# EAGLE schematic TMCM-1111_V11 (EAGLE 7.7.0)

## Sheet 1 of 5: CPU
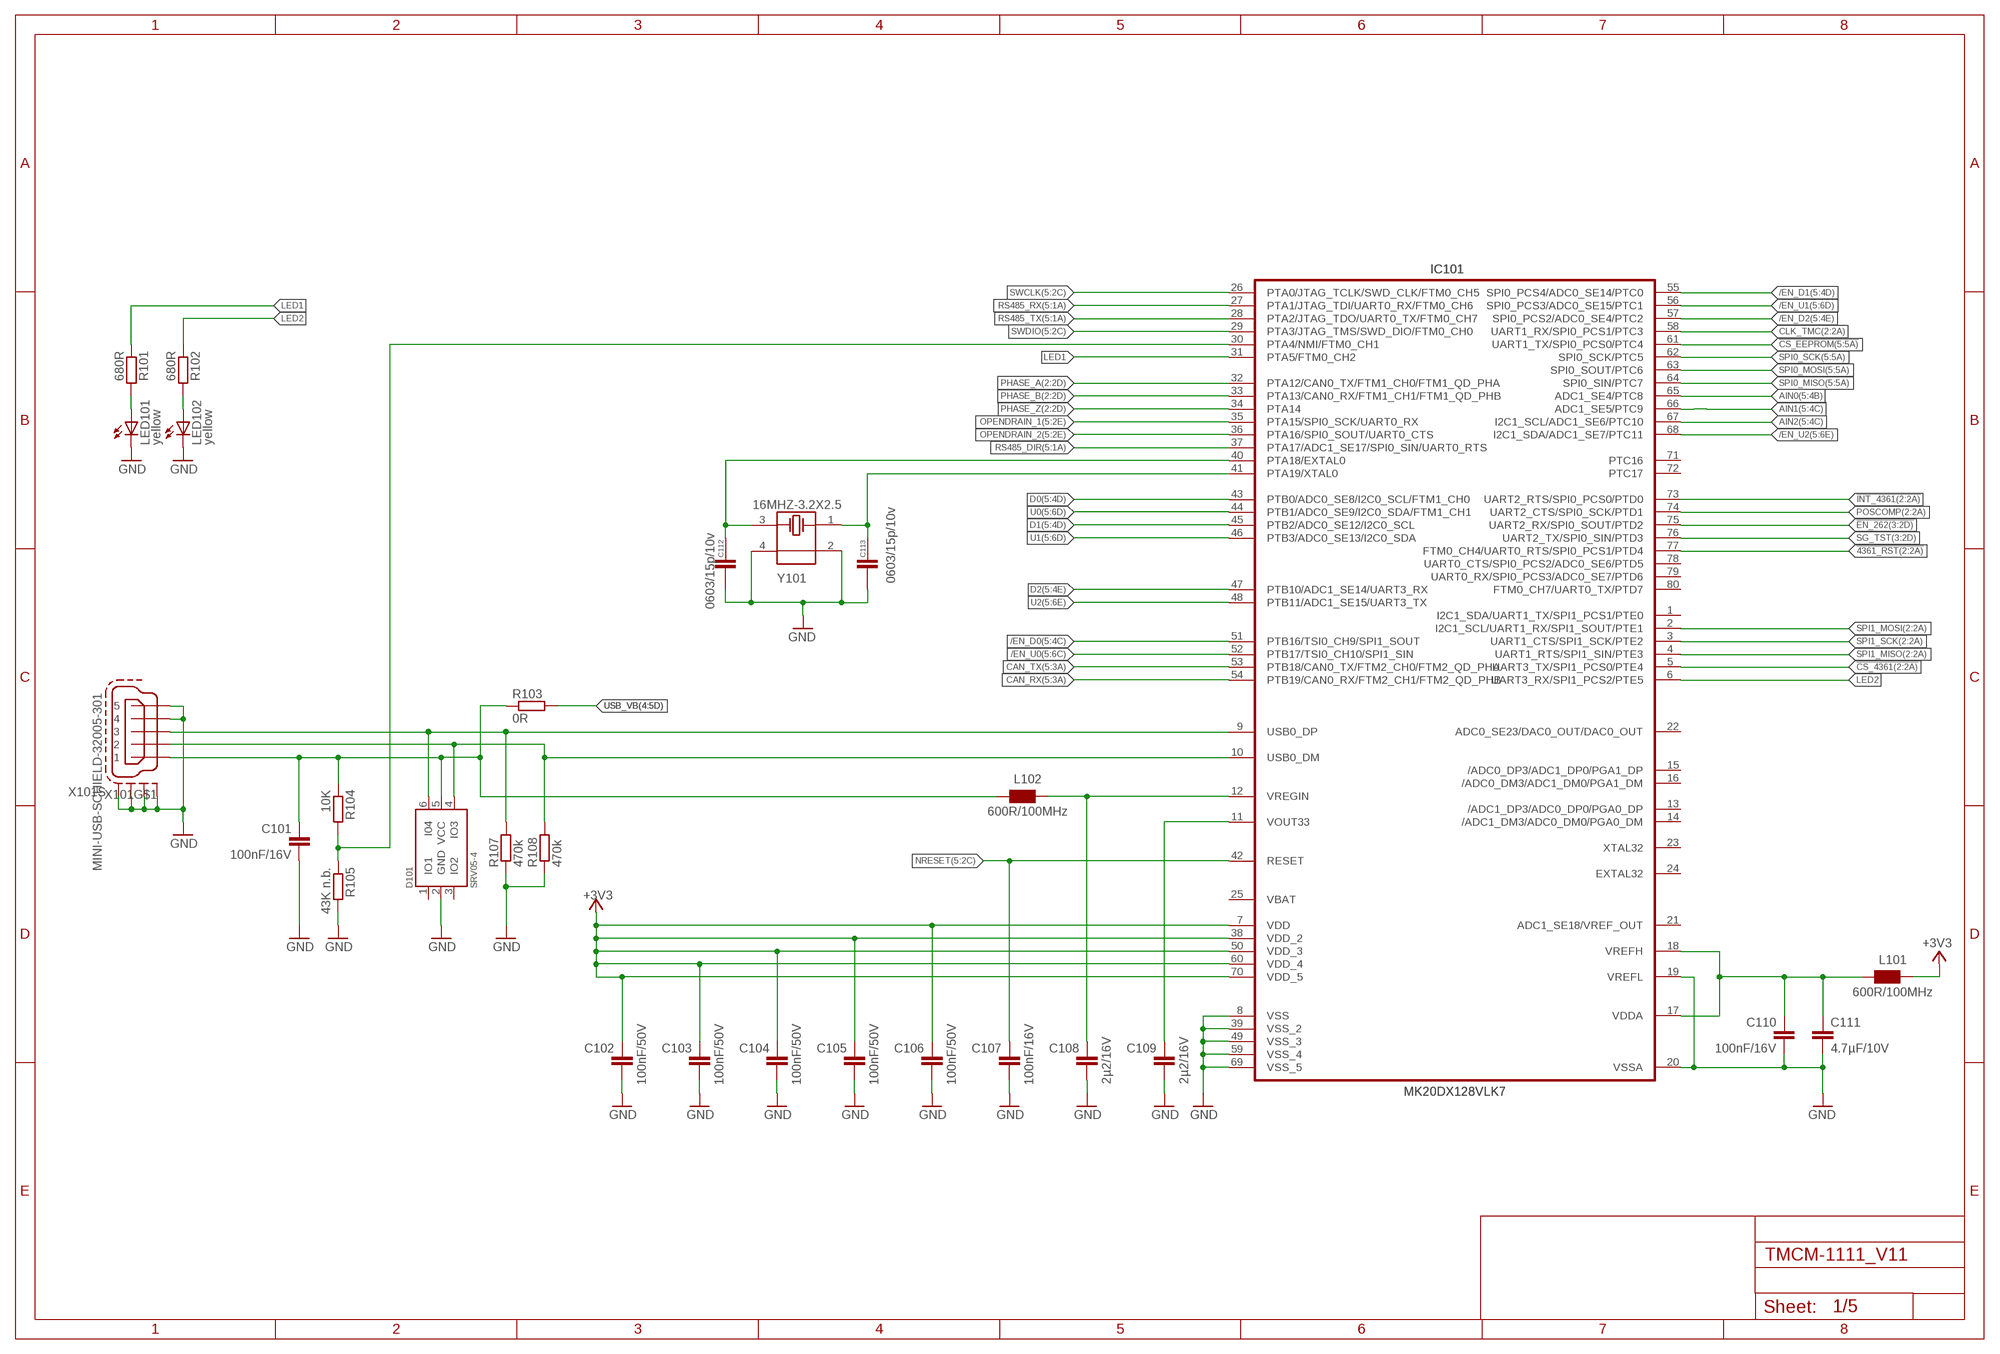
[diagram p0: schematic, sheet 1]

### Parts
C101  100nF/16V  C-EUC0603  [C0603]
C102  100nF/50V  C-EUC0603  [C0603]
C103  100nF/50V  C-EUC0603  [C0603]
C104  100nF/50V  C-EUC0603  [C0603]
C105  100nF/50V  C-EUC0603  [C0603]
C106  100nF/50V  C-EUC0603  [C0603]
C107  100nF/16V  C-EUC0603  [C0603]
C108  2µ2/16V  C-EUC0603  [C0603]
C109  2µ2/16V  C-EUC0603  [C0603]
C110  100nF/16V  C-EUC0603  [C0603]
C111  4.7µF/10V  C-EUC0603  [C0603]
C112  0603/15p/10v  C/0603  [0603]
C113  0603/15p/10v  C/0603  [0603]
D101  SRV05-4  [TMC_SOT23-6]
IC101  MK20DX128VLK7  [LQFP80_12X12X0.5]
L101  600R/100MHz  WE-CBF_0603  [0603]
L102  600R/100MHz  WE-CBF_0603  [0603]
LED101  yellow  LEDCHIP-LED0603  [CHIP-LED0603]
LED102  yellow  LEDCHIP-LED0603  [CHIP-LED0603]
R101  680R  R-EU_R0603  [R0603]
R102  680R  R-EU_R0603  [R0603]
R103  0R  R-EU_R0603  [R0603]
R104  10K  R-EU_R0603  [R0603]
R105  43K n.b.  R-EU_R0603  [R0603]
R107  470k  R-EU_R0603  [R0603]
R108  470k  R-EU_R0603  [R0603]
X101  MINI-USB-SCHIELD-32005-301  [32005-301]
Y101  16MHZ-3.2X2.5  MYLIB_CRYSTAL-16MHZ-3.2X2.5  [MYLIB_FA-238]

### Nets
!4361_RST: IC101.77(FTM0_CH4/UART0_RTS/SPI0_PCS1/PTD4) ; also sheet 2
!CS_4361: IC101.5(UART3_TX/SPI1_PCS0/PTE4) ; also sheet 2
!CS_EEPROM: IC101.61(UART1_TX/SPI0_PCS0/PTC4) ; also sheet 5
!EN_262: IC101.75(UART2_RX/SPI0_SOUT/PTD2) ; also sheet 3
!INT_4361: IC101.73(UART2_RTS/SPI0_PCS0/PTD0) ; also sheet 2
+3V3: C102.1 C103.1 C104.1 C105.1 C106.1 IC101.7(VDD) IC101.38(VDD_2) IC101.50(VDD_3) IC101.60(VDD_4) IC101.70(VDD_5) L101.1 ; also sheet 2,3,4,5
/EN_D0: IC101.51(PTB16/TSI0_CH9/SPI1_SOUT) ; also sheet 5
/EN_D1: IC101.55(SPI0_PCS4/ADC0_SE14/PTC0) ; also sheet 5
/EN_D2: IC101.57(SPI0_PCS2/ADC0_SE4/PTC2) ; also sheet 5
/EN_U0: IC101.52(PTB17/TSI0_CH10/SPI1_SIN) ; also sheet 5
/EN_U1: IC101.56(SPI0_PCS3/ADC0_SE15/PTC1) ; also sheet 5
/EN_U2: IC101.68(I2C1_SDA/ADC1_SE7/PTC11) ; also sheet 5
AIN0: IC101.65(ADC1_SE4/PTC8) ; also sheet 5
AIN1: IC101.66(ADC1_SE5/PTC9) ; also sheet 5
AIN2: IC101.67(I2C1_SCL/ADC1_SE6/PTC10) ; also sheet 5
CAN_RX: IC101.54(PTB19/CAN0_RX/FTM2_CH1/FTM2_QD_PHB) ; also sheet 5
CAN_TX: IC101.53(PTB18/CAN0_TX/FTM2_CH0/FTM2_QD_PHA) ; also sheet 5
CLK_TMC: IC101.58(UART1_RX/SPI0_PCS1/PTC3) ; also sheet 2,3
D0: IC101.43(PTB0/ADC0_SE8/I2C0_SCL/FTM1_CH0) ; also sheet 5
D1: IC101.45(PTB2/ADC0_SE12/I2C0_SCL) ; also sheet 5
D2: IC101.47(PTB10/ADC1_SE14/UART3_RX) ; also sheet 5
GND: C101.2 C102.2 C103.2 C104.2 C105.2 C106.2 C107.2 C108.2 C109.2 C110.2 C111.2 C112.1 C113.1 D101.2(GND) IC101.8(VSS) IC101.19(VREFL) IC101.20(VSSA) IC101.39(VSS_2) IC101.49(VSS_3) IC101.59(VSS_4) IC101.69(VSS_5) LED101.C LED102.C R105.2 R107.1 R108.1 X101.4 X101.5 X101.M1(S:S1) X101.M2(S:S2) X101.M3(S:S3) X101.M4(S:S4) Y101.2 Y101.4 ; also sheet 2,3,4,5
LED1: IC101.31(PTA5/FTM0_CH2) R101.1
LED2: IC101.6(UART3_RX/SPI1_PCS2/PTE5) R102.1
N$18: IC101.30(PTA4/NMI/FTM0_CH1) R104.2 R105.1
N$19: C109.1 IC101.11(VOUT33)
N$21 [GND]: D101.6(I04) IC101.9(USB0_DP) R107.2 X101.3
N$22 [GND]: D101.4(IO3) IC101.10(USB0_DM) R108.2 X101.2
N$23: LED101.A R101.2
N$24: LED102.A R102.2
N$27: C108.1 IC101.12(VREGIN) L102.1
N$31: C112.2 IC101.40(PTA18/EXTAL0) Y101.3
N$33: C113.2 IC101.41(PTA19/XTAL0) Y101.1
NRESET: C107.1 IC101.42(RESET) ; also sheet 5
OPENDRAIN_1: IC101.35(PTA15/SPI0_SCK/UART0_RX) ; also sheet 5
OPENDRAIN_2: IC101.36(PTA16/SPI0_SOUT/UART0_CTS) ; also sheet 5
PHASE_A: IC101.32(PTA12/CAN0_TX/FTM1_CH0/FTM1_QD_PHA) ; also sheet 2,5
PHASE_B: IC101.33(PTA13/CAN0_RX/FTM1_CH1/FTM1_QD_PHB) ; also sheet 2,5
PHASE_Z: IC101.34(PTA14) ; also sheet 2,5
POSCOMP: IC101.74(UART2_CTS/SPI0_SCK/PTD1) ; also sheet 2
RS485_DIR: IC101.37(PTA17/ADC1_SE17/SPI0_SIN/UART0_RTS) ; also sheet 5
RS485_RX: IC101.27(PTA1/JTAG_TDI/UART0_RX/FTM0_CH6) ; also sheet 5
RS485_TX: IC101.28(PTA2/JTAG_TDO/UART0_TX/FTM0_CH7) ; also sheet 5
SG_TST: IC101.76(UART2_TX/SPI0_SIN/PTD3) ; also sheet 3
SPI0_MISO: IC101.64(SPI0_SIN/PTC7) ; also sheet 5
SPI0_MOSI: IC101.63(SPI0_SOUT/PTC6) ; also sheet 5
SPI0_SCK: IC101.62(SPI0_SCK/PTC5) ; also sheet 5
SPI1_MISO: IC101.4(UART1_RTS/SPI1_SIN/PTE3) ; also sheet 2
SPI1_MOSI: IC101.2(I2C1_SCL/UART1_RX/SPI1_SOUT/PTE1) ; also sheet 2
SPI1_SCK: IC101.3(UART1_CTS/SPI1_SCK/PTE2) ; also sheet 2
SWCLK: IC101.26(PTA0/JTAG_TCLK/SWD_CLK/FTM0_CH5) ; also sheet 5
SWDIO: IC101.29(PTA3/JTAG_TMS/SWD_DIO/FTM0_CH0) ; also sheet 5
U0: IC101.44(PTB1/ADC0_SE9/I2C0_SDA/FTM1_CH1) ; also sheet 5
U1: IC101.46(PTB3/ADC0_SE13/I2C0_SDA) ; also sheet 5
U2: IC101.48(PTB11/ADC1_SE15/UART3_TX) ; also sheet 5
USB_VB: R103.2 ; also sheet 4
USB_VBUS: C101.1 D101.5(VCC) L102.2 R103.1 R104.1 X101.1
VDDA: C110.1 C111.1 IC101.17(VDDA) IC101.18(VREFH) L101.2
Unconnected: D101.1(IO1) D101.3(IO2) IC101.1(I2C1_SDA/UART1_TX/SPI1_PCS1/PTE0) IC101.13(/ADC1_DP3/ADC0_DP0/PGA0_DP) IC101.14(/ADC1_DM3/ADC0_DM0/PGA0_DM) IC101.15(/ADC0_DP3/ADC1_DP0/PGA1_DP) IC101.16(/ADC0_DM3/ADC1_DM0/PGA1_DM) IC101.21(ADC1_SE18/VREF_OUT) IC101.22(ADC0_SE23/DAC0_OUT/DAC0_OUT) IC101.23(XTAL32) IC101.24(EXTAL32) IC101.71(PTC16) IC101.72(PTC17) IC101.78(UART0_CTS/SPI0_PCS2/ADC0_SE6/PTD5) IC101.79(UART0_RX/SPI0_PCS3/ADC0_SE7/PTD6) IC101.80(FTM0_CH7/UART0_TX/PTD7)

## Sheet 2 of 5: TMC-429
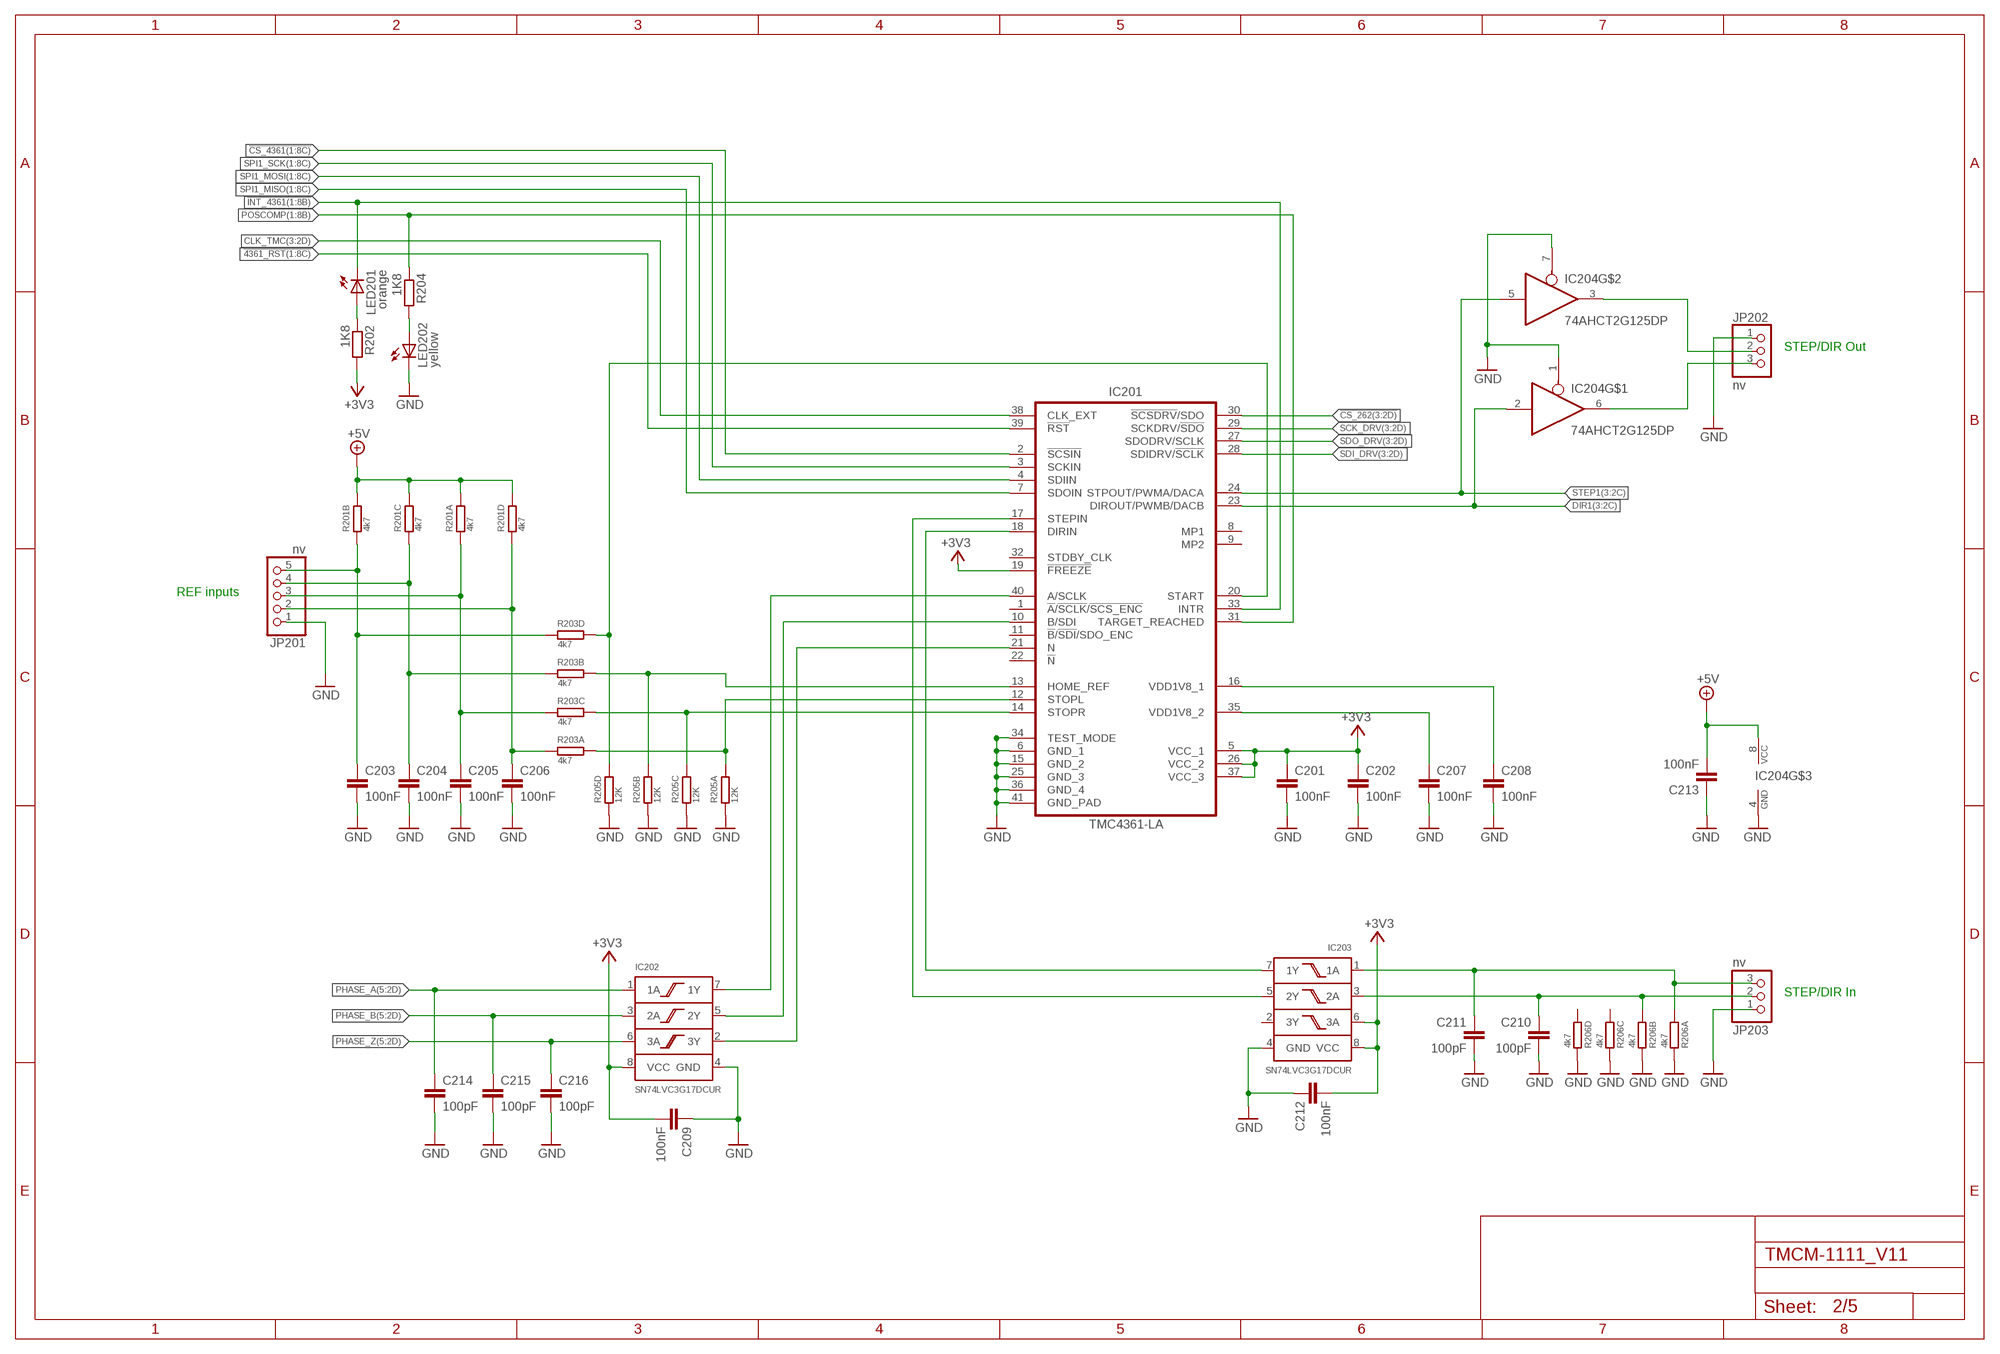
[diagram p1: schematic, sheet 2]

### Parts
C201  100nF  C-EUC0603  [C0603]
C202  100nF  C-EUC0603  [C0603]
C203  100nF  C-EUC0603  [C0603]
C204  100nF  C-EUC0603  [C0603]
C205  100nF  C-EUC0603  [C0603]
C206  100nF  C-EUC0603  [C0603]
C207  100nF  C-EUC0603  [C0603]
C208  100nF  C-EUC0603  [C0603]
C209  100nF  C-EUC0603  [C0603]
C210  100pF  C-EUC0603  [C0603]
C211  100pF  C-EUC0603  [C0603]
C212  100nF  C-EUC0603  [C0603]
C213  100nF  C-EUC0603  [C0603]
C214  100pF  C-EUC0603  [C0603]
C215  100pF  C-EUC0603  [C0603]
C216  100pF  C-EUC0603  [C0603]
IC201  TMC4361-LA  TMC4361-LA  [TMC_QFN40_0.5_6.0X6.0]
IC202  SN74LVC3G17DCUR  [US8_DCU]
IC203  SN74LVC3G17DCUR  [US8_DCU]
IC204  74AHCT2G125DP  74AHCT2G125DCT  [SSOP08]
JP201  nv  PINHD-1X5  [1X05]
JP202  nv  PINHD-1X3  [1X03]
JP203  nv  PINHD-1X3  [1X03]
LED201  orange  LEDCHIP-LED0603  [CHIP-LED0603]
LED202  yellow  LEDCHIP-LED0603  [CHIP-LED0603]
R201  4k7  R_NET_4X  [R_4X_1206]
R202  1K8  R-EU_R0603  [R0603]
R203  4k7  R_NET_4X  [R_4X_1206]
R204  1K8  R-EU_R0603  [R0603]
R205  12K  R_NET_4X  [R_4X_1206]
R206  4k7  R_NET_4X  [R_4X_1206]

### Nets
!4361_RST: IC201.39(!RST!) ; also sheet 1
!CS_262: IC201.30(!SCSDRV!/SDO) ; also sheet 3
!CS_4361: IC201.2(!SCSIN!) ; also sheet 1
!INT_4361: IC201.33(INTR) LED201.C ; also sheet 1
+3V3: C201.1 C202.1 C209.2 C212.2 IC201.5(VCC_1) IC201.19(!FREEZE!) IC201.26(VCC_2) IC201.37(VCC_3) IC202.8(VCC) IC203.6(3A) IC203.8(VCC) R202.2 ; also sheet 1,3,4,5
+5V: C213.2 IC204.8(VCC) R201.P$5 R201.P$6 R201.P$7 R201.P$8 ; also sheet 4,5
CLK_TMC: IC201.38(CLK_EXT) ; also sheet 1,3
DIR1: IC201.23(DIROUT/PWMB/DACB) IC204.2(I) ; also sheet 3
GND: C201.2 C202.2 C203.2 C204.2 C205.2 C206.2 C207.2 C208.2 C209.1 C210.2 C211.2 C212.1 C213.1 C214.2 C215.2 C216.2 IC201.6(GND_1) IC201.15(GND_2) IC201.25(GND_3) IC201.34(TEST_MODE) IC201.36(GND_4) IC201.41(GND_PAD) IC202.4(GND) IC203.4(GND) IC204.1(OE) IC204.4(GND) IC204.7(OE) JP201.1 JP202.1 JP203.1 LED202.C R205.P$1 R205.P$2 R205.P$3 R205.P$4 R206.P$1 R206.P$2 R206.P$3 R206.P$4 ; also sheet 1,3,4,5
N$15: LED202.A R204.2
N$16: LED201.A R202.1
N$20: IC201.12(STOPL) R203.P$8 R205.P$8
N$25: C208.1 IC201.16(VDD1V8_1)
N$26: C207.1 IC201.35(VDD1V8_2)
N$30: IC201.14(STOPR) R203.P$6 R205.P$6
N$32: IC201.13(HOME_REF) R203.P$7 R205.P$7
N$36: IC201.40(A/SCLK) IC202.7(1Y)
N$37: IC201.18(DIRIN) IC203.7(1Y)
N$44: IC201.20(START) R203.P$5 R205.P$5
N$45: IC201.10(B/SDI) IC202.5(2Y)
N$46: IC204.3(O) JP202.2
N$47: IC201.21(N) IC202.2(3Y)
N$48: IC204.6(O) JP202.3
N$49: IC201.17(STEPIN) IC203.5(2Y)
N$51: C210.1 IC203.3(2A) JP203.2 R206.P$7
N$52: C211.1 IC203.1(1A) JP203.3 R206.P$8
PHASE_A: C214.1 IC202.1(1A) ; also sheet 1,5
PHASE_B: C215.1 IC202.3(2A) ; also sheet 1,5
PHASE_Z: C216.1 IC202.6(3A) ; also sheet 1,5
POSCOMP: IC201.31(TARGET_REACHED) R204.1 ; also sheet 1
REF1: C206.1 JP201.2 R201.P$4 R203.P$1
REF2: C204.1 JP201.4 R201.P$3 R203.P$2
REFR1: C205.1 JP201.3 R201.P$1 R203.P$3
REFR2: C203.1 JP201.5 R201.P$2 R203.P$4
SCK_DRV: IC201.29(SCKDRV/!SDO!) ; also sheet 3
SDI_DRV: IC201.28(SDIDRV/!SCLK!) ; also sheet 3
SDO_DRV: IC201.27(SDODRV/SCLK) ; also sheet 3
SPI1_MISO: IC201.7(SDOIN) ; also sheet 1
SPI1_MOSI: IC201.4(SDIIN) ; also sheet 1
SPI1_SCK: IC201.3(SCKIN) ; also sheet 1
STEP1: IC201.24(STPOUT/PWMA/DACA) IC204.5(I) ; also sheet 3
Unconnected: IC201.1(!A!/!SCLK!/!SCS_ENC) IC201.8(MP1) IC201.9(MP2) IC201.11(!B!/!SDI!/SDO_ENC) IC201.22(!N!) IC201.32(STDBY_CLK) IC203.2(3Y) R206.P$5 R206.P$6

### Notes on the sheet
- STEP/DIR Out
- REF inputs
- STEP/DIR In

## Sheet 3 of 5: DRIVER
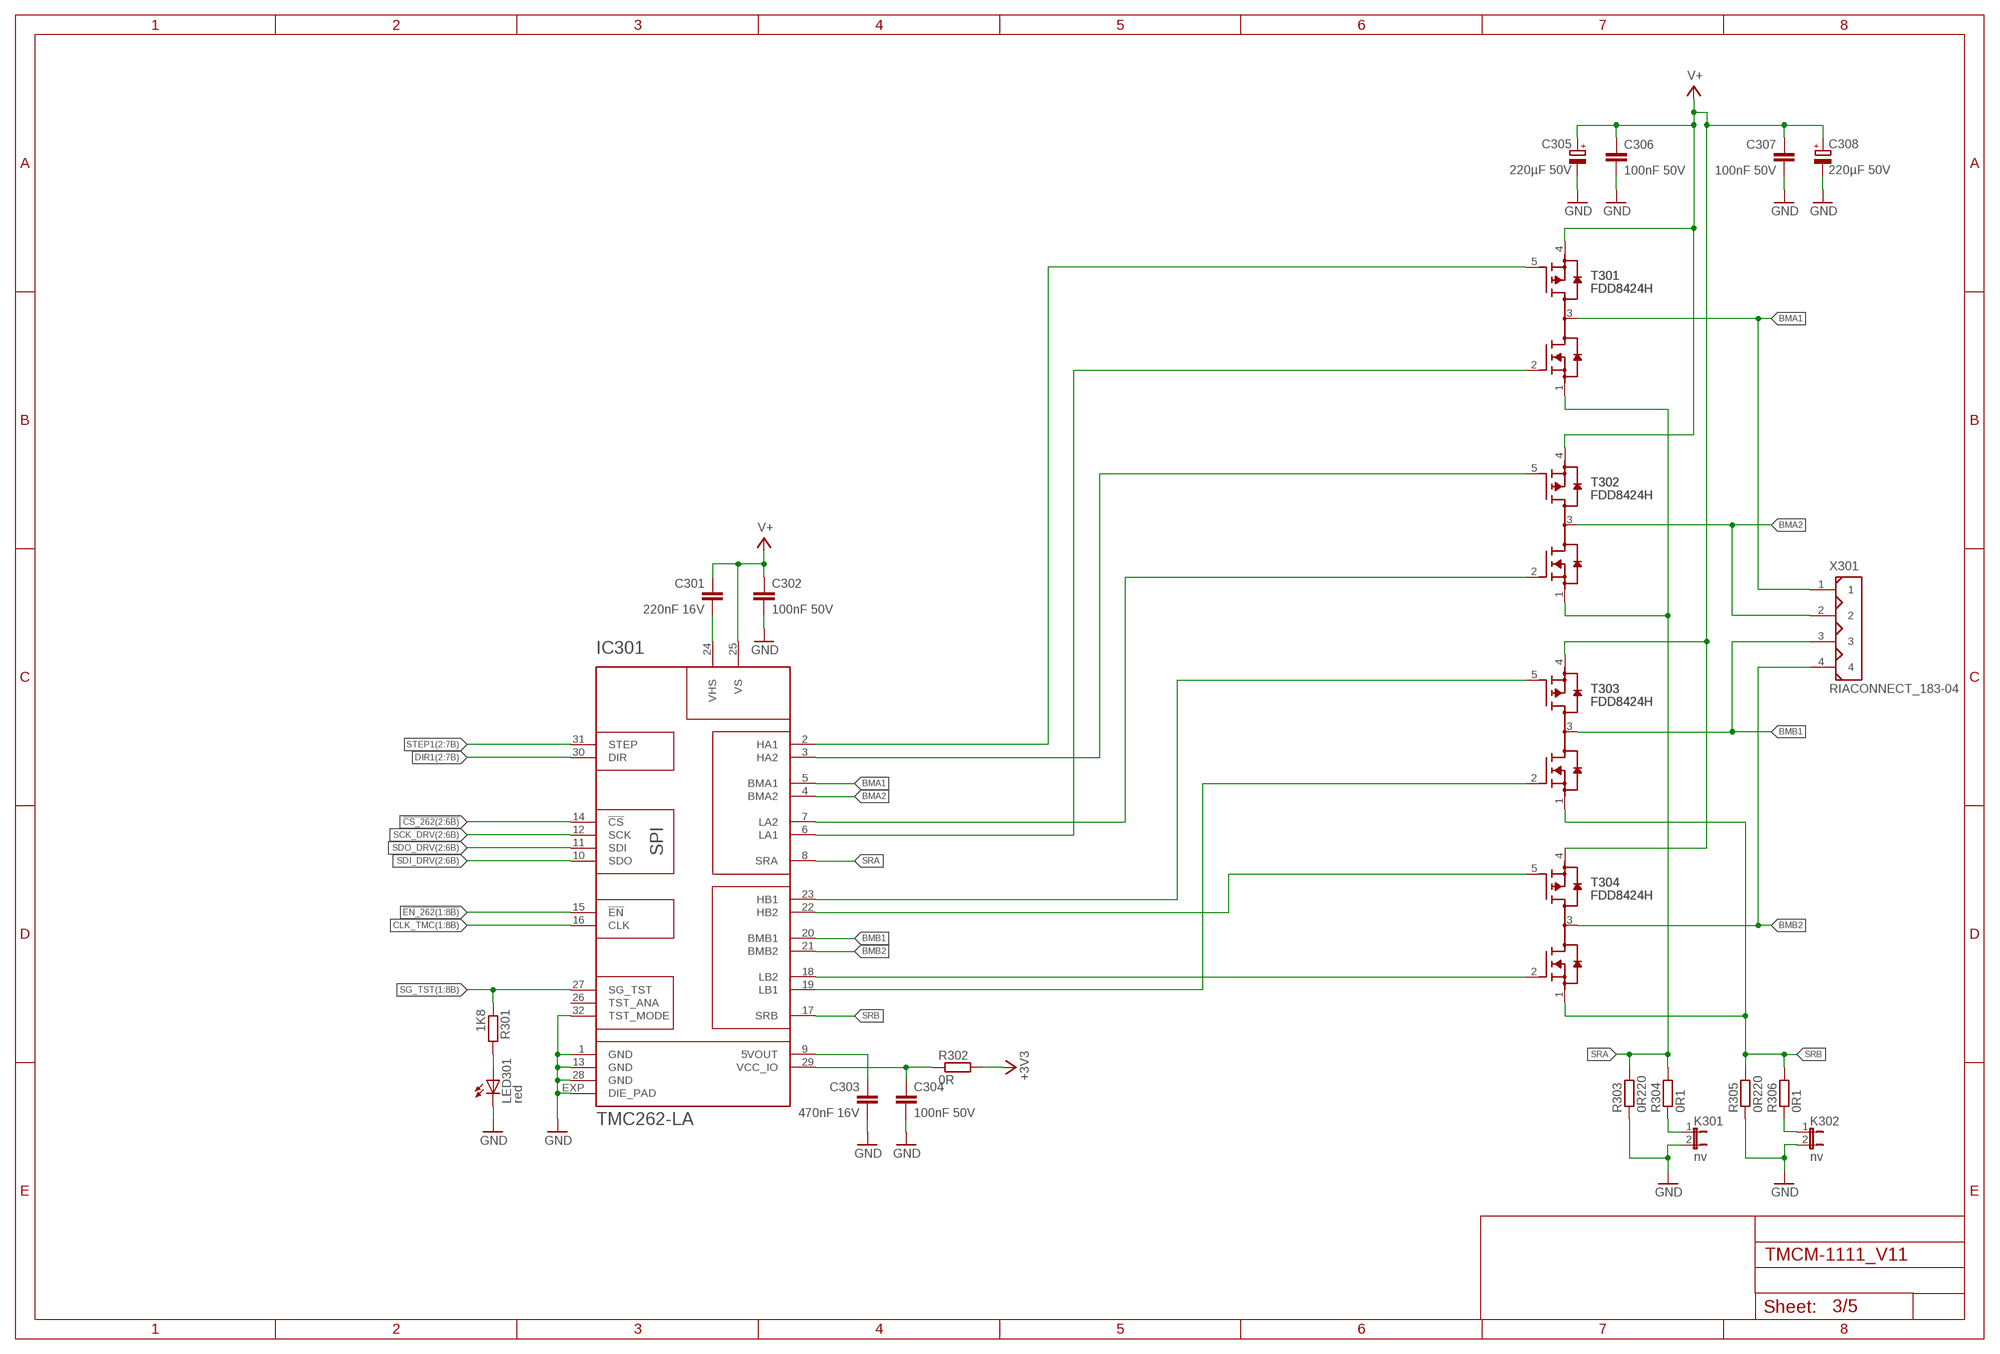
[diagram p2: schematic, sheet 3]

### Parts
C301  220nF 16V  C-EUC0603  [C0603]
C302  100nF 50V  C-EUC0603  [C0603]
C303  470nF 16V  C-EUC0603  [C0603]
C304  100nF 50V  C-EUC0603  [C0603]
C305  220µF 50V  CPOL-EUE5-10.5  [E5-10,5]
C306  100nF 50V  C-EUC0603  [C0603]
C307  100nF 50V  C-EUC0603  [C0603]
C308  220µF 50V  CPOL-EUE5-10.5  [E5-10,5]
IC301  TMC262-LA  [QFN32_5X5]
K301  nv  JP1E  [JP1]
K302  nv  JP1E  [JP1]
LED301  red  LEDCHIP-LED0603  [CHIP-LED0603]
R301  1K8  R-EU_R0603  [R0603]
R302  0R  R-EU_R0603  [R0603]
R303  0R220  R-EU_R1206  [R1206]
R304  0R1  R-EU_R1206  [R1206]
R305  0R220  R-EU_R1206  [R1206]
R306  0R1  R-EU_R1206  [R1206]
T301  FDD8424H  [DUAL_DPAK_4L]
T302  FDD8424H  [DUAL_DPAK_4L]
T303  FDD8424H  [DUAL_DPAK_4L]
T304  FDD8424H  [DUAL_DPAK_4L]
X301  RIACONNECT_183-04  [RIACONNECT_183-04]

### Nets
!CS_262: IC301.14(!CS) ; also sheet 2
!EN_262: IC301.15(!EN) ; also sheet 1
+3V3: R302.2 ; also sheet 1,2,4,5
BMA1: IC301.5(BMA1) T301.3(D_NP) X301.1
BMA2: IC301.4(BMA2) T302.3(D_NP) X301.2
BMB1: IC301.20(BMB1) T303.3(D_NP) X301.3
BMB2: IC301.21(BMB2) T304.3(D_NP) X301.4
CLK_TMC: IC301.16(CLK) ; also sheet 1,2
DIR1: IC301.30(DIR) ; also sheet 2
GND: C302.2 C303.2 C304.2 C305.- C306.2 C307.2 C308.- IC301.1(GND) IC301.13(GND) IC301.28(GND) IC301.32(TST_MODE) IC301.EXP(DIE_PAD) K301.2 K302.2 LED301.C R303.1 R305.1 ; also sheet 1,2,4,5
N$1: LED301.A R301.2
N$2: C304.1 IC301.29(VCC_IO) R302.1
N$3: C303.1 IC301.9(5VOUT)
N$4: C301.2 IC301.24(VHS)
N$5: IC301.2(HA1) T301.5(G_P)
N$6: IC301.3(HA2) T302.5(G_P)
N$7: IC301.7(LA2) T302.2(G_N)
N$8: IC301.6(LA1) T301.2(G_N)
N$9: IC301.23(HB1) T303.5(G_P)
N$10: IC301.22(HB2) T304.5(G_P)
N$11: IC301.19(LB1) T303.2(G_N)
N$12: IC301.18(LB2) T304.2(G_N)
N$13: K302.1 R306.1
N$14: K301.1 R304.1
SCK_DRV: IC301.12(SCK) ; also sheet 2
SDI_DRV: IC301.10(SDO) ; also sheet 2
SDO_DRV: IC301.11(SDI) ; also sheet 2
SG_TST: IC301.27(SG_TST) R301.1 ; also sheet 1
SRA: IC301.8(SRA) R303.2 R304.2 T301.1(S_N) T302.1(S_N)
SRB: IC301.17(SRB) R305.2 R306.2 T303.1(S_N) T304.1(S_N)
STEP1: IC301.31(STEP) ; also sheet 2
V+: C301.1 C302.1 C305.+ C306.1 C307.1 C308.+ IC301.25(VS) T301.4(S_P) T302.4(S_P) T303.4(S_P) T304.4(S_P) ; also sheet 4,5
Unconnected: IC301.26(TST_ANA)

## Sheet 4 of 5: SUPPLY
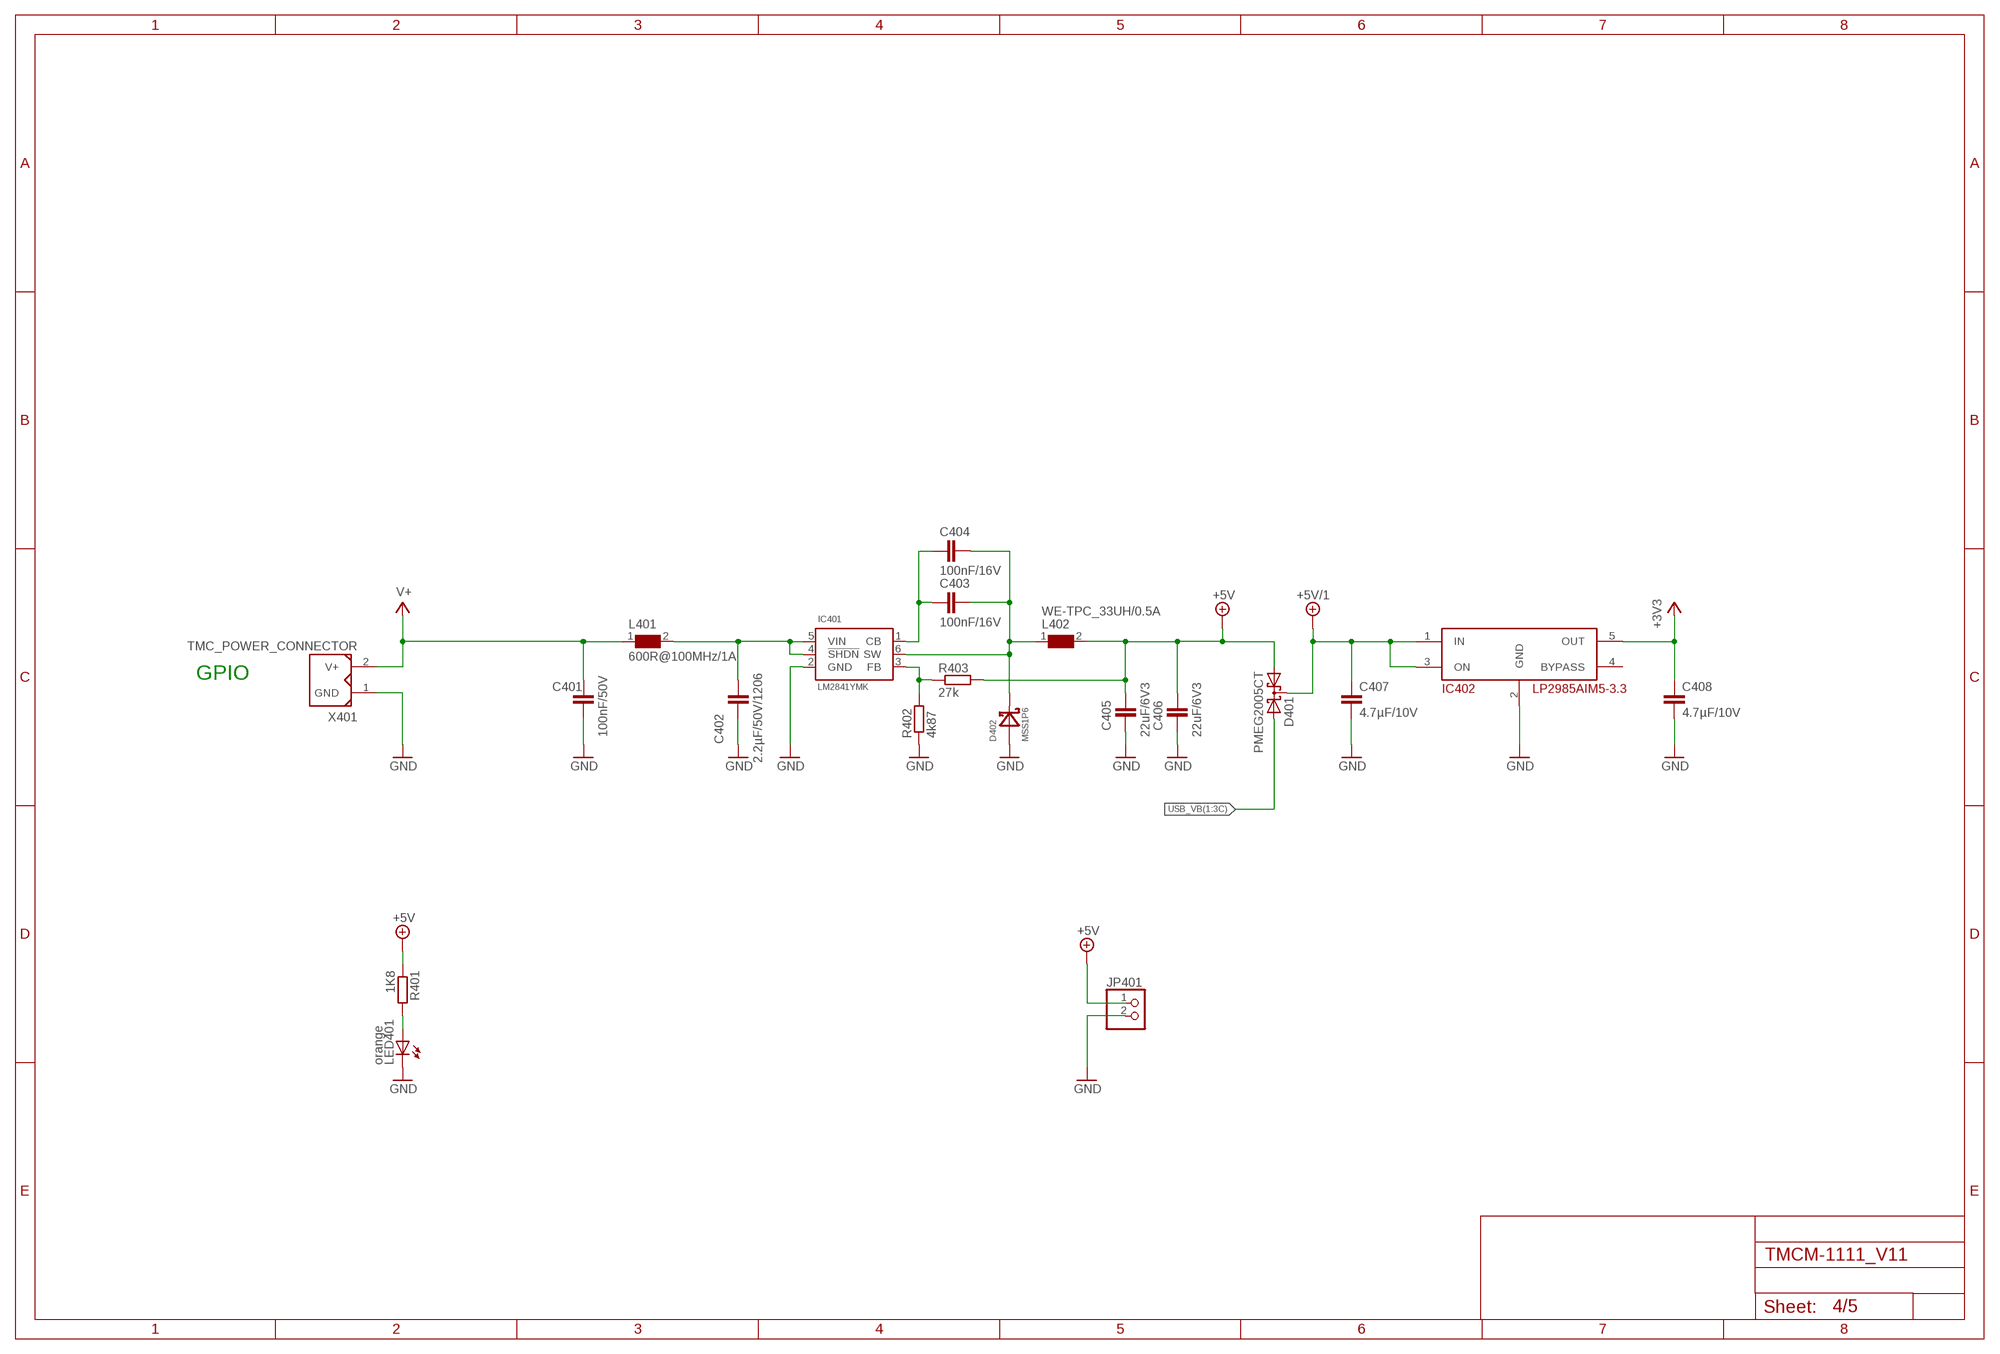
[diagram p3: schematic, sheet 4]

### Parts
C401  100nF/50V  C-EUC0603  [C0603]
C402  2.2µF/50V/1206  C-EUC1206  [C1206]
C403  100nF/16V  C-EUC0603  [C0603]
C404  100nF/16V  C-EUC0603  [C0603]
C405  22uF/6V3  C-EUC0805  [C0805]
C406  22uF/6V3  C-EUC0805  [C0805]
C407  4.7µF/10V  C-EUC0603  [C0603]
C408  4.7µF/10V  C-EUC0603  [C0603]
D401  PMEG2005CT  [SOT23]
D402  MSS1P6  [MICRO_SMP]
IC401  LM2841YMK  [TMC_SOT23-6]
IC402  LP2985AIM5-3.3  [SOT23-5]
JP401  PINHD-1X2  [1X02]
L401  600R@100MHz/1A  WE-CBF_0603  [0603]
L402  WE-TPC_33UH/0.5A  [WE-TPC_4818/4828]
LED401  orange  LEDCHIP-LED0603  [CHIP-LED0603]
R401  1K8  R-EU_R0603  [R0603]
R402  4k87  R-EU_R0603  [R0603]
R403  27k  R-EU_R0603  [R0603]
X401  TMC_POWER_CONNECTOR  [RIACONNECT_320-02]

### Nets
+3V3: C408.1 IC402.5(OUT) ; also sheet 1,2,3,5
+5V: C405.1 C406.1 D401.1(A1) JP401.1 L402.2 R401.1 R403.2 ; also sheet 2,5
+5V/1: C407.1 D401.3(C) IC402.1(IN) IC402.3(ON)
GND: C401.2 C402.2 C405.2 C406.2 C407.2 C408.2 D402.A IC401.2(GND) IC402.2(GND) JP401.2 LED401.C R402.1 X401.1(GND) ; also sheet 1,2,3,5
N$17: C402.1 IC401.4(!SHDN) IC401.5(VIN) L401.2
N$34: C403.1 C404.1 IC401.1(CB)
N$35: C403.2 C404.2 D402.C IC401.6(SW) L402.1
N$38: LED401.A R401.2
N$40: IC401.3(FB) R402.2 R403.1
USB_VB: D401.2(A2) ; also sheet 1
V+: C401.1 L401.1 X401.2(V+) ; also sheet 3,5
Unconnected: IC402.4(BYPASS)

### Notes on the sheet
- GPIO

## Sheet 5 of 5: MISC
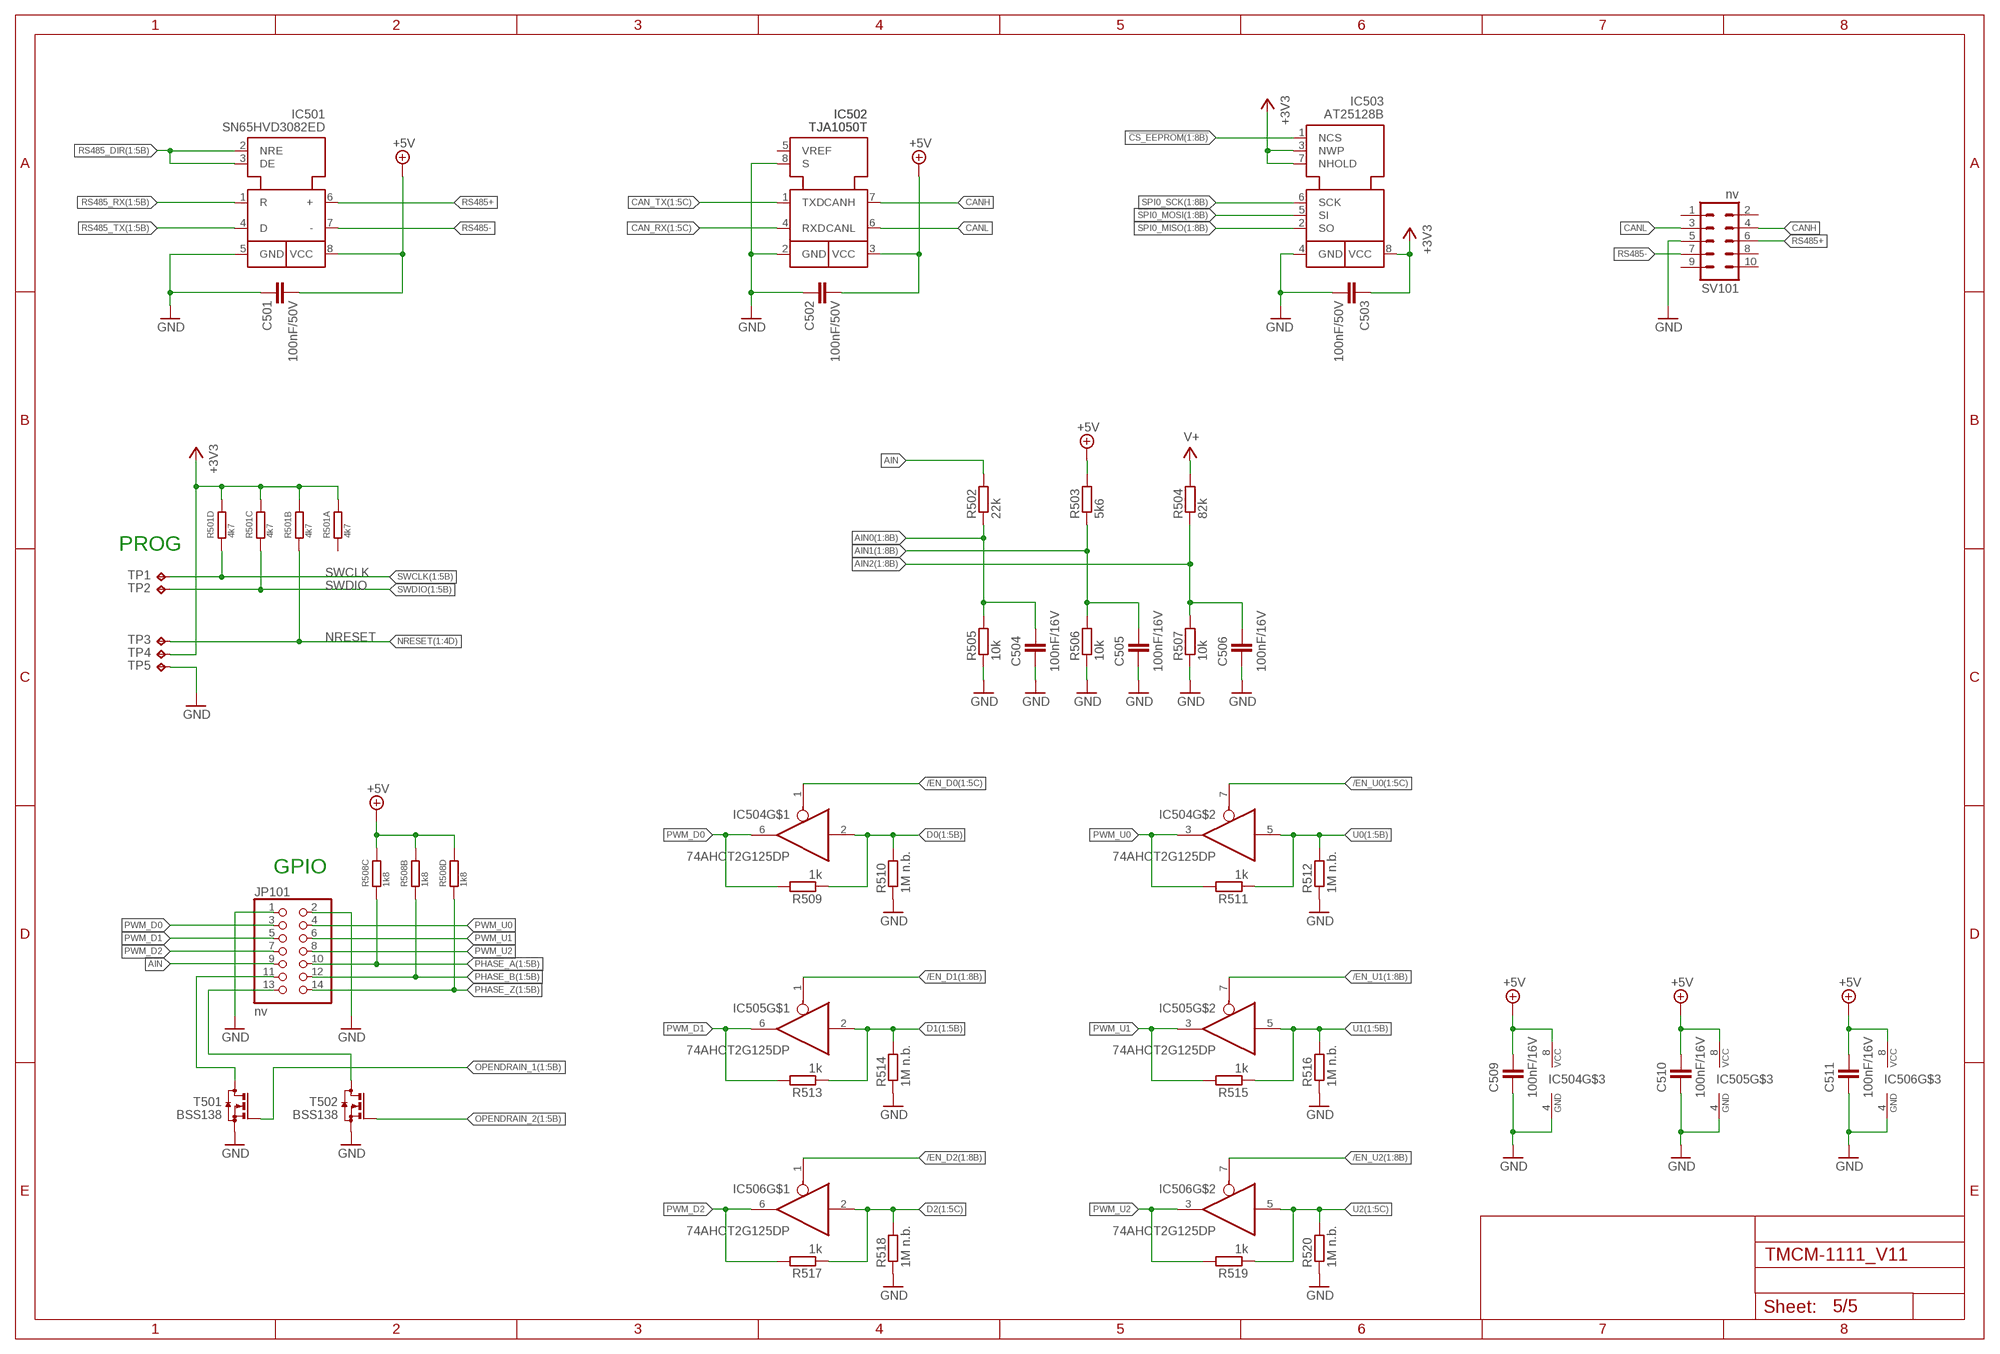
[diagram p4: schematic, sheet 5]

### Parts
C501  100nF/50V  C-EUC0603  [C0603]
C502  100nF/50V  C-EUC0603  [C0603]
C503  100nF/50V  C-EUC0603  [C0603]
C504  100nF/16V  C-EUC0603  [C0603]
C505  100nF/16V  C-EUC0603  [C0603]
C506  100nF/16V  C-EUC0603  [C0603]
C509  100nF/16V  C-EUC0603  [C0603]
C510  100nF/16V  C-EUC0603  [C0603]
C511  100nF/16V  C-EUC0603  [C0603]
IC501  SN65HVD3082ED  [SO8]
IC502  TJA1050T  [SO8]
IC503  AT25128B  [SO8]
IC504  74AHCT2G125DP  74AHCT2G125DCT  [SSOP08]
IC505  74AHCT2G125DP  74AHCT2G125DCT  [SSOP08]
IC506  74AHCT2G125DP  74AHCT2G125DCT  [SSOP08]
JP101  nv  PINHD-2X7  [2X07]
R501  4k7  R_NET_4X  [R_4X_1206]
R502  22k  R-EU_R0603  [R0603]
R503  5k6  R-EU_R0603  [R0603]
R504  82k  R-EU_R0603  [R0603]
R505  10k  R-EU_R0603  [R0603]
R506  10k  R-EU_R0603  [R0603]
R507  10k  R-EU_R0603  [R0603]
R508  1k8  R_NET_4X  [R_4X_1206]
R509  1k  R-EU_R0603  [R0603]
R510  1M n.b.  R-EU_R0603  [R0603]
R511  1k  R-EU_R0603  [R0603]
R512  1M n.b.  R-EU_R0603  [R0603]
R513  1k  R-EU_R0603  [R0603]
R514  1M n.b.  R-EU_R0603  [R0603]
R515  1k  R-EU_R0603  [R0603]
R516  1M n.b.  R-EU_R0603  [R0603]
R517  1k  R-EU_R0603  [R0603]
R518  1M n.b.  R-EU_R0603  [R0603]
R519  1k  R-EU_R0603  [R0603]
R520  1M n.b.  R-EU_R0603  [R0603]
SV101  nv  ML10  [ML10]
T501  BSS138  [SOT23]
T502  BSS138  [SOT23]
TP1  TPTP15SQ  [TP15SQ]
TP2  TPTP15SQ  [TP15SQ]
TP3  TPTP15SQ  [TP15SQ]
TP4  TPTP15SQ  [TP15SQ]
TP5  TPTP15SQ  [TP15SQ]

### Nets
!CS_EEPROM: IC503.1(NCS) ; also sheet 1
+3V3: C503.1 IC503.3(NWP) IC503.7(NHOLD) IC503.8(VCC) R501.P$5 R501.P$6 R501.P$7 R501.P$8 TP4.TP ; also sheet 1,2,3,4
+5V: C501.2 C502.2 C509.1 C510.1 C511.1 IC501.8(VCC) IC502.3(VCC) IC504.8(VCC) IC505.8(VCC) IC506.8(VCC) R503.2 R508.P$5 R508.P$6 R508.P$7 ; also sheet 2,4
/EN_D0: IC504.1(OE) ; also sheet 1
/EN_D1: IC505.1(OE) ; also sheet 1
/EN_D2: IC506.1(OE) ; also sheet 1
/EN_U0: IC504.7(OE) ; also sheet 1
/EN_U1: IC505.7(OE) ; also sheet 1
/EN_U2: IC506.7(OE) ; also sheet 1
AIN: JP101.9 R502.2
AIN0: C504.1 R502.1 R505.2 ; also sheet 1
AIN1: C505.1 R503.1 R506.2 ; also sheet 1
AIN2: C506.1 R504.1 R507.2 ; also sheet 1
CAN_RX: IC502.4(RXD) ; also sheet 1
CAN_TX: IC502.1(TXD) ; also sheet 1
CANH: IC502.7(CANH) SV101.4
CANL: IC502.6(CANL) SV101.3
D0: IC504.2(I) R509.1 R510.2 ; also sheet 1
D1: IC505.2(I) R513.1 R514.2 ; also sheet 1
D2: IC506.2(I) R517.1 R518.2 ; also sheet 1
GND: C501.1 C502.1 C503.2 C504.2 C505.2 C506.2 C509.2 C510.2 C511.2 IC501.5(GND) IC502.2(GND) IC502.8(S) IC503.4(GND) IC504.4(GND) IC505.4(GND) IC506.4(GND) JP101.1 JP101.2 R505.1 R506.1 R507.1 R510.1 R512.1 R514.1 R516.1 R518.1 R520.1 SV101.5 T501.2(S) T502.2(S) TP5.TP ; also sheet 1,2,3,4
N$55: JP101.13 T502.3(D)
N$56: JP101.11 T501.3(D)
NRESET: R501.P$2 TP3.TP ; also sheet 1
OPENDRAIN_1: T501.1(G) ; also sheet 1
OPENDRAIN_2: T502.1(G) ; also sheet 1
PHASE_A: JP101.10 R508.P$3 ; also sheet 1,2
PHASE_B: JP101.12 R508.P$2 ; also sheet 1,2
PHASE_Z: JP101.14 R508.P$4 ; also sheet 1,2
PWM_D0: IC504.6(O) JP101.3 R509.2
PWM_D1: IC505.6(O) JP101.5 R513.2
PWM_D2: IC506.6(O) JP101.7 R517.2
PWM_U0: IC504.3(O) JP101.4 R511.2
PWM_U1: IC505.3(O) JP101.6 R515.2
PWM_U2: IC506.3(O) JP101.8 R519.2
RS485+: IC501.6(+) SV101.6
RS485-: IC501.7(-) SV101.7
RS485_DIR: IC501.2(NRE) IC501.3(DE) ; also sheet 1
RS485_RX: IC501.1(R) ; also sheet 1
RS485_TX: IC501.4(D) ; also sheet 1
SPI0_MISO: IC503.2(SO) ; also sheet 1
SPI0_MOSI: IC503.5(SI) ; also sheet 1
SPI0_SCK: IC503.6(SCK) ; also sheet 1
SWCLK: R501.P$4 TP1.TP ; also sheet 1
SWDIO: R501.P$3 TP2.TP ; also sheet 1
U0: IC504.5(I) R511.1 R512.2 ; also sheet 1
U1: IC505.5(I) R515.1 R516.2 ; also sheet 1
U2: IC506.5(I) R519.1 R520.2 ; also sheet 1
V+: R504.2 ; also sheet 3,4
Unconnected: IC502.5(VREF) R501.P$1 R508.P$1 R508.P$8 SV101.1 SV101.2 SV101.8 SV101.9 SV101.10

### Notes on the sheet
- PROG
- GPIO

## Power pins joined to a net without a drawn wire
VBAT: IC101.25(VBAT)

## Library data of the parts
C101-C111 C201-C216 C301-C304 C306 C307 C401-C404 C407 C408 C501-C506 C509-C511 = rcl:C-EU: CAPACITOR, European symbol
C112 C113 = _TMC_TE_RCL:C
C305 C308 = rcl:CPOL-EU: POLARIZED CAPACITOR, European symbol
C405 C406 = rcl:C-EU: CAPACITOR, European symbol; HERSTELLER: KEMET; HERST_NR: C0805C226M9PAC7800
D101 = TMC_IC:SRV05-4
D401 = diode:PMEG2005CT: MEGA Schottky Diodes 500mA lowVf dual MEGA Schottky barrier rectifier
D402 = Dioden:MSS1P6: SMT Schottky Barrier Rectifier 1A / 60V
IC101 = NemoParts:MK20DX128VLK7: Kinetis K 32-bit MCU, ARM Cortex-M4 core, 128KB Flash, 72MHz, USB, QFP 80; BESCHREIBUNG: Kinetis K 32-bit MCU, ARM Cortex-M4 core, 128KB Flash, 72MHz, USB, QFP 80; BEST-NR1: MK20DX128VLK7; GEOMETRY_HEIGHT: 1,6mm; HERSTELLER1: NXP/Freescale; WERT: MK20DX128VLK7
IC201 = TMCM-1110_V30:TMC4361-LA: S-ramp motion controller for stepper motors with high velocities. With SPI and Step/Dir; QFN40(5x5); DESCRIPTION: S-ramp motion controller for stepper motors with high velocities_ With SPI and Step/Dir; QFN40(5x5); DISTRIBUTOR1: Digi-Key; GEOMETRY_HEIGHT: 0,9mm; MANUFACTURER: TRINAMIC; ORDERCODE-DISTRI1: 1460-1131-1-ND; ORDERCODE-MANU1: TMC4361-LA
IC202 IC203 = TMC4670_DEV_v11:SN74LVC3G17DCUR
IC204 IC504-IC506 = NemoParts:74*2G125: Dual line drivers with 3-state outputs.
IC301 = stepRocker:TMC262-LA: TRINAMIC Energy efficient microstep driver for external MOSFET's for up to 6A with coolStep&trade; Information given in this library is believed to be accurate and reliable. However no warranty is given for its correctness. Datasheet for TMC260/261/262 Description Energy efficient microstep driver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
IC401 = TMC_IC:LM2841YMK: 300mA/600 mA up to 42V Input Step-Down DC/DC Regulator in Thin SOT-23
IC402 = stepRocker:LP2985AIM5-3.3
IC501 = stepRocker:SN65HVD3082ED: RS484-Transceiver
IC502 = NemoParts:TJA1050T: CAN-Transceive
IC503 = stepRocker:AT25128B
JP101 = pinhead:PINHD-2X7: PIN HEADER
JP201 = TMC4670_DEV_v11:PINHD-1X5: PIN HEADER
JP202 JP203 = pinhead:PINHD-1X3: PIN HEADER
JP401 = NemoParts:PINHD-1X2: PIN HEADER
K301 K302 = jumper:JP1E: JUMPER
L101 L102 = wuerth-elektronik:WE-CBF: SMD EMI Suppression Ferrite Beads
L401 = Wuerth_Elektronik_eiSos_V6:WE-CBF: SMD EMI Suppression Ferrite Beads WE-CBF; HERSTELLER: Würth; HERST_NR: 742792651
L402 = NemoParts:WE-TPC_33UH/0.5A: Shielded Tiny Power Inductor WE-TPC; BEST-NR-LIEF: 2082509; BEST-NR1: 744042330; HERSTELLER1: Wuerth; LIEFERANT: Farnell
LED101 LED102 LED201 LED202 LED301 LED401 = led:LED: LED
R101-R105 R107 R108 R202 R204 R301-R306 R401-R403 R502-R507 R509-R520 = rcl:R-EU_: RESISTOR, European symbol
R201 R203 R205 R206 R501 R508 = stepRocker:R_NET_4X
SV101 = con-harting-ml:ML10: HARTING; OC_FARNELL: unknown; OC_NEWARK: unknown
T301-T304 = NemoParts:FDD8424H: Dual N & P-Channel 60V Power MOSFET with low on-resistance and fast switching performance High energy efficiency and good thermal performance
T501 T502 = Transistoren:BSS138: N-CHANNEL MOS FET
TP1-TP5 = testpad:TP: Test pad
X101 = con-cypressindustries:MINI-USB-SCHIELD-: MINI USB-B Conector Source: www.cypressindustries.com; OC_FARNELL: unknown; OC_NEWARK: unknown
X301 = stepRocker:RIACONNECT_183-04
X401 = stepRocker:TMC_POWER_CONNECTOR
Y101 = EBC_ucBoard_TE_v04:MYLIB_CRYSTAL-16MHZ-3.2X2.5

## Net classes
0 default: clearance 0.15 mm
